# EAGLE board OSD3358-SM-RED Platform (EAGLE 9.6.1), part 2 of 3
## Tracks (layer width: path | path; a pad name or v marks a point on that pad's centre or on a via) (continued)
GND  (via drill 0.3, 0.3 pad 0.61, 0.5) (continued)
  Top 0.254: S1.4 S1.2 | S2.3 S2.1 | R37.2 v7.72,47.12 | R38.2 v7.72,49.02 | R35.2 v7.72,43.31 | R36.2 v7.72,45.21 | R26.2 v7.72,41.27 | X4.4 X4.8 | U14.4 17.53,7.42 17.37,7.26 v17.2,7.26 | U13.4 15.12,7.37 14.99,7.24 v14.61,7.24 | U11.4 18.79,15.38 18.92,15.24 R100.2 | C61.2 R100.2 | R100.2 v20.02,15.98 | C74.2 19.48,18.72 19.41,18.8 U12.4 | U12.4 | U12.4 18.79,18.29 18.67,18.16 v17.2,18.16 | C41.2 v21.79,16.64 | C40.2 v29.01,16.64 | C46.2 v25.43,22.12 | C2.1 70.32,10.93 v69.98,10.59 69.55,10.16 C1.1 | R59.1 R58.1 R56.1 R57.1 v81.56,46.43 | R65.1 R64.1 R63.1 R62.1 R61.1 R60.1 v86.54,45.54 | R66.1 R67.1 R68.1 v95.78,46.43 | R55.1 81.69,42.37 v81.25,42.37 | R54.1 R53.1 v83.19,45.06 | U10.61 U10.62 U10.63 87.05,41.17 v86.97,41.1 v91.59,41.1 91.55,41.14 U10.54 U10.53 | C14.2 C54.2 C59.2 96.11,28.78 v96.83,28.78 | R115.2 v26.04,35.56 | C57.2 C55.2 | C52.2 85.27,33.38 85.83,32.82 v85.93,32.72 | C62.2 v19.68,8.64 | v100.64,24.77 J4.8 | J4.10 v100.64,26.04 | J4.12 v100.64,27.3 | J4.16 v100.64,29.84 | J4.20 v100.64,32.38 | v100.64,22.23 J4.4 | C39.2 v93.12,27.03 93.12,27.48 93.03,27.57 Y3.2 | U7.N2 76.48,39.59 v76.48,38.43 | U7.G5 73.48,41.22 73.97,41.71 v74.37,41.71 | U7.J5 74.49,41.59 v74.37,41.71 | U7.E7 72.64,42.09 73.13,42.57 v73.13,42.98 73.56,42.98 73.99,43.41 U7.H10 | U7.K8 74.88,42.6 74.37,42.09 v74.37,41.71 | U7.A6 70.45,41.63 v69.47,41.63 | C91.2 85.83,24.61 v85.83,25.15 85.83,25.96 C89.2 | U22.9 U22.8 80.86,24.78 80.85,24.79 v79.88,24.79 79.4,24.79 C92.2 | v79.88,26.31 80.74,26.31 80.78,26.27 U22.5 | v82.78,26.57 82.73,26.52 82.45,26.52 82.2,26.27 U22.3
  Top 0.305: C93.2 v43.1,15.04 | v10.85,41.88 11.07,41.66 C3.2 | C51.2 v21.59,6.22 | U21.4 v38.48,10.54 | R39.1 v105.54,18.41 | C57.2 v96.83,30.86 | C21.2 95.38,17.65 v93.85,17.65 | C79.2 C88.2 v78.61,13.59
  Top 0.381: C22.2 v102.31,11.3 | C63.2 33.25,15.21 v33.86,15.21
  Top 0.762: D2.A 40.64,48.18 41.27,48.82 J5.1 | C11.- v35.56,36.35
  Bottom 0.152: R141.1 26.87,16.26 v26.49,15.88 | C13.1 v71.25,36.52 | X6.5 103.3,39.12 103.63,39.45 105.89,39.45 v106.05,39.29 | v103.66,40.59 103.45,40.59 103.18,40.32 X6.8 | X6.2 105.56,37.92 v106.07,38.43 | X6.16 100.5,38.52 v100.48,38.53 | v99.77,41 100,40.77 100,40.41 100.69,39.72 X6.13 | R18.1 54.86,27.91 55.09,27.69 v55.63,27.69 | 27.13,33.71 C77.2 C64.2 | C68.2 v24.92,27.05 | R1.2 43.54,35.03 v43.28,35.28 | C43.2 76.33,17.4 v76.58,17.14 | U2.4 10.42,47.02 v11.12,47.02 | U15.TH 25.04,18.69 v25.04,18.67 | v90.09,28.91 89.15,28.91 89.14,28.91 88.61,28.91 88.5,29.02 U25.1 | v55.63,26.42 55.3,26.75 R16.1
  Bottom 0.203: C75.2 v34.37,34.42 | C65.2 28.4,32.08 27.48,32.99 v27.1,32.99 | C78.2 v27.1,35.43 | C53.2 83.9,33.33 83.62,33.05 v83.62,32.82
  Bottom 0.254: v69.98,10.59 70.88,11.49 U6.1 72.38,11.49 72.67,11.79 R27.1 73.56,11.79 73.66,11.68 73.66,10.79 73.79,10.67 C6.1 | U6.4 74.05,9.99 74.22,10.16 C6.1 | C20.1 C18.1 73.28,48.11 73.43,48.26 v73.79,48.26 74.14,48.26 74.3,48.11 C19.1 | C35.2 C36.2 C37.2 C38.2 v80.85,31.55 | C34.2 C28.2 C27.2 | C27.2 C26.2 | C26.2 C25.2 | C32.2 C33.2 v86.97,41.1 C23.2 85.8,41.1 85.09,41.81 v85.09,42.6 | C31.2 C30.2 v91.59,41.1 92.35,41.1 C29.2 | C26.2 80.31,39.37 80.26,39.32 C24.2 79.86,39.29 v79.86,38.56 80.06,38.35 C27.2 | C77.2 C78.2 | C66.2 C67.2 25.98,32.74 26.24,32.99 v27.1,32.99 27.1,33.68 27.13,33.71 | C6.1 v74.98,10.67 | C17.1 75.41,41.71 v74.37,41.71 | C90.1 87.5,24.03 v88.06,24.59
  Bottom 0.305: R113.1 23.62,9.4 v24.13,9.91 | C16.1 v65.66,44.88 | X3.6 91.76,17.65 v93.85,17.65 | X3.GND 102.1,13.59 v101.22,13.59 | C101.2 C100.2 26.24,14.81 26.49,15.06 v26.49,15.88 | v24.89,10.67 24.89,9.65 24.64,9.4 C42.2 C99.2 | C50.2 26.67,9.45 26.21,9.91 v25.65,9.91 | 27.69,9.91 v27.18,9.91 | R112.1 27.69,9.91 | v27.18,11.43 27.74,10.87 C49.2 | R111.1 27.89,9.7 27.69,9.91
  Bottom 0.381: X1.GND v5.43,47.98 v5.44,47.98 | U15.1 28.66,20.02 28.83,20.19 28.83,20.83 v28.57,21.08 | v34.42,26.82 C76.2 C72.2 | v35.56,26.82 C70.2 C71.2
  other vias: 25.65,11.43 30.1,29.21 90.3,37.82 28.98,30.61 30.1,30.61 31.22,30.61 28.98,29.21 31.22,29.21 28.98,27.81 31.22,27.81 24.13,12.95 25.65,12.95 27.18,12.95 24.89,12.19 26.42,12.19 24.13,11.43 26.42,10.67 55.63,30.1 60.58,30.23 63.12,30.1 65.51,30.07 55.5,25.15 55.63,22.61 55.63,20.19 58.04,20.19 63.12,20.19 65.53,20.19 65.53,22.61 65.66,25.15 65.53,27.69 88.14,40.01 89.15,40.01 90.3,40.01 91.31,40.01 92.33,40.01 88.14,38.99 89.15,38.99 90.3,38.99 91.31,38.99 92.33,38.99 88.14,37.85 89.15,37.85 91.31,37.85 92.33,37.85 88.14,36.7 89.15,36.7 90.3,36.7 91.31,36.7 92.33,36.7 88.14,35.69 89.15,35.69 90.3,35.69 91.31,35.69 92.33,35.69 30.1,27.81 25.04,19.43 25.81,19.43 25.81,18.67 33.86,15.98 86.79,32.69 99.19,36.83 99.24,40.36 85.17,37.82 80.85,29.77 60.58,20.19 48.16,41 48.16,38.89 49.23,37.8 43.56,37.97 19.05,47.5 19.05,48.39 19.05,46.61 24,48.39 24,47.5 24,46.61 59.74,42.52 59.74,41.76 56.77,20.19 59.31,20.19 61.85,20.19 64.26,20.19 65.53,23.88 61.85,30.1 64.39,30.1
  pour Route2: -3.81,58.42 111.76,58.42 111.76,-3.81 -3.81,-3.81
  pour Top (rank 6): 55.5,20.07 59.31,20.07 59.31,19.43 61.85,19.43 61.85,20.07 65.66,20.07 65.66,23.88 66.29,23.88 66.29,26.42 65.66,26.42 65.66,30.23 61.85,30.23 61.85,30.86 59.31,30.86 59.31,30.23 55.5,30.23 55.5,26.42 54.86,26.42 54.86,23.88 56.13,23.88 56.13,29.59 65.02,29.59 65.02,20.7 56.13,20.7 56.13,23.24 55.5,23.24
  pour Top (rank 6): 55.5,23.24 55.5,23.88 56.13,23.88 56.13,23.24
  pour Top: 19.94,45.09 17.78,47.24 15.88,47.24 15.37,46.74 13.59,46.74 13.21,47.12 13.21,48.39 17.91,48.39 18.41,48.9 24.13,48.9 24.77,48.26 24.77,45.72 24.13,45.09
  pour Top (no thermals): 85.6,34.16 87.25,34.16 87.63,33.78 87.63,32.72 87.05,32.13 85.47,32.13 85.22,32.38 85.22,33.66
  pour Top (no thermals): 85.72,38.3 86.39,38.3 86.39,37.41 84.84,37.41 84.84,38.3
  pour Top (no thermals): 86.87,42.57 88.24,42.57 88.24,40.64 87,40.64 86.87,40.64 86.56,40.94 86.56,41.48 86.87,41.78
  pour Top (no thermals): 91.72,42.57 92.28,42.57 92.28,40.64 91.29,40.64 91.29,42.57
  pour Bottom (no thermals): 81.38,29.31 80.62,29.31 80.62,30.18 81.41,30.18 81.41,31.22 80.62,31.22 80.62,31.8 82.04,31.8 82.04,29.87 81.94,29.87
  pour Bottom (no thermals): 30.35,16.76 34.16,16.76 34.16,13.59 31.11,13.59 31.11,14.61 30.35,14.61
  pour Top (no thermals): 96.85,40.31 98.78,40.31 99.14,40.67 99.62,40.67 99.62,40.11 98.6,40.11 98.42,39.93 96.85,39.93
  pour Top (no thermals): 96.88,37.24 99.69,37.19 99.69,36.53 99.14,36.53 98.91,36.83 96.88,36.83
  pour Top (no thermals): 89,28.5 89,29.51 90.4,29.51 90.4,28.24 89.76,28.24 89.76,29.21 89.76,29.24 89.26,29.24 89.26,28.5
  pour Top (rank 2, no thermals): 50.14,39.62 48.46,39.62 48.46,38.56 49.53,38.56 49.53,37.64 50.29,37.64 50.29,36.73 49.07,36.73 49.07,38.1 48.16,38.1 47.7,38.71 47.7,41.76 48.46,41.76 48.46,40.23 50.14,40.23
  pour Top (rank 2, no thermals): 43.18,38.73 44.83,38.73 44.83,37.21 43.18,37.21
  pour Bottom: 18.54,48.64 24.38,48.64 24.38,45.09 18.54,45.09
  pour Top (no thermals): 57.91,42.82 61.72,42.82 61.72,41.45 57.91,41.45
GPIO0_7  (via drill 0.3)
  Top 0.152: v79.27,15.04 79.07,15.24 R9.2 77.98,15.24 77.85,15.37 77.85,16.64 v77.34,17.14
  Bottom 0.152: v79.27,15.04 79.88,14.43 80.97,14.43 84.58,10.82 84.58,9.75 85.5,8.84 85.5,6.86 86.56,5.79 90.73,5.79 J6.42 | R2.2 76.66,18.49 77.34,17.8 v77.34,17.14
GPIO0_7SRC  (via drill 0.3)
  Top 0.152: U1.C5 64.59,18.16 64.39,17.96 v64.39,17.3
  Bottom 0.152: v64.39,17.3 64.39,17.02 64.62,16.79 65.15,16.79 65.89,17.53 71.07,17.53 72.03,18.49 R2.1
GPIO0_26  (via drill 0.3)
  Top 0.152: U1.R5 65.02,33.96 65.51,34.44 65.51,35.36 64.77,36.09 64.77,45.97 62.69,48.06 62.69,50.8 62.48,51 v62.48,51.44
  Bottom 0.152: J5.14 56.52,51.94 56.87,51.59 61.9,51.59 62.05,51.44 v62.48,51.44
GPIO0_27
  Top 0.152: U1.T5 65.02,35.41 64.47,35.97 64.47,45.85 61.59,48.72 J5.17
GPIO1_12
  Top 0.152: U1.P6 63.75,32.64 62.97,33.43 62.97,35.31 62.94,35.33 62.94,45.21 61.52,46.63 60.07,46.63 58.24,48.46 54.13,48.46 52.91,49.68 52.91,51.64 J5.12
GPIO1_13
  Top 0.152: U1.R6 63.27,33.88 63.27,35.43 63.25,35.46 63.25,45.34 61.65,46.94 60.2,46.94 58.37,48.77 55.37,48.77 J5.11
GPIO1_14
  Top 0.152: U1.T6 63.75,35.38 63.55,35.59 63.55,45.47 61.77,47.24 60.33,47.24 57.96,49.61 57.96,51.61 J5.16
GPIO1_15
  Top 0.152: U1.P7 62.97,31.65 63.96,31.65 64.24,31.93 64.24,35.33 63.86,35.71 63.86,45.59 61.9,47.55 60.45,47.55 59.05,48.95 J5.15
GPIO1_16
  Bottom 0.152: R14.2 R23.2 56.03,32.26 55.78,32 55.02,32 53.24,30.23 52.88,30.23 52.4,29.74 52.4,24.28 50.37,22.25 50.37,15.34 52.83,12.88 52.83,7.11 53.7,6.25 58.83,6.25 60.2,4.88 60.2,3.05 J6.15
GPIO1_17  (via drill 0.3)
  Top 0.152: U1.R12 56.13,32.82 56.62,32.33 56.62,31.93 56.16,31.47 v55.75,31.47
  Bottom 0.152: v55.75,31.47 54.91,31.47 53.37,29.92 53.01,29.92 52.7,29.62 52.7,24.16 50.67,22.12 50.67,15.47 53.14,13.01 53.14,7.24 53.82,6.55 58.95,6.55 60.5,5 60.5,3.5 60.96,3.05 62.2,3.05 62.87,2.39 62.87,1.27 63.3,0.84 68.15,0.84 J6.23
GPIO1_28  (via drill 0.3)
  Top 0.152: U1.N14 53.59,31.45 53.44,31.6 v52.98,31.6
  Bottom 0.152: v52.98,31.6 52.96,31.6 51.49,30.12 51.49,24.66 49.45,22.63 49.45,14.96 51.92,12.5 51.92,6.5 J6.12
GPIO1_29  (via drill 0.3)
  Top 0.152: U1.P3 68.15,32.13 68.63,32.61 70.43,32.61 73.28,35.46 v73.28,35.97
  Bottom 0.152: v73.28,35.97 73.28,38.84 69.98,42.14 69.98,44.55 69.32,45.21 69.32,45.87 69.47,46.02 69.47,47.99 70.64,49.16 70.64,52.48 70.87,52.7 J5.26
GPIO2_1  (via drill 0.3)
  Top 0.152: U1.T7 62.48,35.36 62.64,35.51 62.64,44.96 61.27,46.33 59.89,46.33 58.67,47.55 v58.06,47.55
  Bottom 0.152: v58.06,47.55 62.15,47.55 63.07,48.46 63.07,52.22 62.59,52.7 J5.18
GPIO3_18  (via drill 0.3)
  Top 0.152: U1.A3 67.67,15.62 68.68,14.61 69.57,14.61 70.21,13.97 v70.21,13.64 | R9.1 77.29,14.71 77.03,14.44 73.6,14.44 73.38,14.22 v73.18,14.22
  Bottom 0.152: v70.21,13.64 70.41,13.44 72.36,13.44 73.15,14.22 v73.18,14.22
GPIO3_19
  Top 0.152: U1.B3 67.56,16.33 68.05,15.85 68.05,15.72 68.83,14.94 69.67,14.94 71.12,13.49 71.12,9.09 70.56,8.53 70.56,6.55 71.32,5.79 72.54,5.79 73.15,5.18 73.15,3.05 J6.27
GPIO3_20
  Top 0.152: R7.1 69.47,13.99 69.16,14.3 68.56,14.3 67.77,15.09 67.41,15.09 67.08,15.42 67.08,17.17 67.56,17.65 U1.C3
GPIO3_21
  Top 0.152: R114.2 72.39,15.44 72.14,15.7 72.14,16.54 71.3,17.37 68.43,17.37 68.05,17.75 68.05,18.52 67.82,18.75 67.26,18.75 66.67,18.16 U1.C4 65.89,18.16 65.66,17.93 65.66,15.47 66.62,14.5 66.62,11.15 66.42,10.95 66.42,9.53 66.95,8.99 69.37,8.99 70.26,8.1 70.26,6.4 71.17,5.49 72.39,5.49 72.85,5.03 72.85,3 J6.25
HDMI_CEC  (via drill 0.3)
  Top 0.152: U10.30 93.05,33.17 93.8,32.41 94.61,32.41 v95.35,31.67 94.59,31.67 93.65,30.73 93.65,25.25 93.07,24.67 D11.C
  Bottom 0.152: X6.12 100.73,40.12 100.31,40.54 100.31,41.78 99.9,42.19 98.15,42.19 97.79,41.83 97.79,32.56 97.43,32.21 95.89,32.21 v95.35,31.67
HDMI_CEC_D
  Top 0.152: R140.2 94.08,23.39 93.11,22.42 D11.A
HDMI_CLK_INH  (via drill 0.3)
  Top 0.152: v88.9,19.43 88.9,20.07 88.29,20.68 88.29,23.04 88.95,23.7 89.94,23.7 90.7,24.46 90.7,26.82 90.91,27.03 R110.1 91.26,28.19 Y3.1 | v88.54,12.5 88.54,11.89 87.94,11.28 86.59,11.28 85.95,10.64 85.95,8.23 85.34,7.62 J7.1
  Bottom 0.152: v88.9,19.43 88.88,19.41 88.88,12.83 v88.54,12.5
HDMI_DSCL  (via drill 0.3)
  Top 0.152: U10.33 94.65,33.77 95.15,33.27 96.39,33.27 96.57,33.1 v96.95,33.1 | v99.34,42.72 98.63,43.43 98.63,44.6 v98.83,44.81
  Bottom 0.152: v96.95,33.1 97.13,33.27 97.13,33.68 97.48,34.04 97.48,42.6 98.15,43.26 99.62,43.26 100.13,42.75 | X6.11 100.76,40.52 100.61,40.66 100.61,42.27 100.38,42.49 | 100.38,42.49 100.13,42.75 | 100.38,42.49 100.13,42.49 | 100.13,42.49 99.57,42.49 v99.34,42.72 | R147.1 97.46,45.49 97.74,45.21 98.65,45.21 98.83,45.03 v98.83,44.81 | 100.13,42.75 100.13,42.49
HDMI_DSDA  (via drill 0.3)
  Top 0.152: U10.32 94.47,33.47 95.2,32.74 v96.09,32.74
  Bottom 0.152: v96.09,32.74 96.32,32.74 96.39,32.82 96.39,33.38 97.18,34.16 97.18,42.72 98.02,43.56 99.47,43.56 | X6.9 102.11,40.72 102.06,40.77 102.06,41.12 101.85,41.33 101.85,41.88 101.68,42.06 101.24,42.06 99.75,43.56 99.64,43.56 | 99.64,43.56 99.47,43.56 | R148.1 98.42,46.1 99.69,44.83 99.69,43.79 | 99.69,43.79 99.69,43.61 99.64,43.56 | 99.47,43.56 99.69,43.79
HDMI_HPD  (via drill 0.3)
  Top 0.152: U10.31 93.55,33.12 93.95,32.72 94.79,32.72 95.07,32.44 95.45,32.44 v96.22,31.67
  Bottom 0.152: X6.19 100.51,37.32 100.25,37.06 99.97,37.06 99.75,36.83 99.75,36.47 99.57,36.3 98.42,36.3 98.2,36.07 98.2,32.44 97.43,31.67 v96.22,31.67
HDMI_INT  (via drill 0.3, 0.3 pad 0.61)
  Top 0.152: U10.50 93.55,42.59 94.08,43.13 96.09,43.13 96.5,43.54 R130.1 96.5,46.89 96.39,46.99 95.91,46.99 95.78,47.12 95.78,48.59 96.09,48.9 97.54,48.9 98.22,49.58 98.22,51.08 v97.99,51.31 | U1.T15 52.02,34.67 v51.69,35 | v75.54,35.97 76.05,35.97 76.53,36.45 77.19,36.45 79.02,38.28 79.02,41.53 78,42.55 78,51.31 v77.78,51.54
  Bottom 0.152: v77.78,51.54 97.77,51.54 v97.99,51.31 | v75.54,35.97 75.54,34.09 75.87,33.76 71.14,29.03 69.27,29.03 68.89,28.65 67.69,28.65 65.23,31.11 65.23,32.03 62.33,34.92 58.85,34.92 58.42,35.36 58.42,36.52 56.59,38.35 51.71,38.35 51.51,38.15 51.51,35.18 v51.69,35
HDMI_SWING
  Top 0.152: U10.34 95.53,34.57 95.71,34.39 95.71,34.19 95.91,33.98 R136.2
HDMI_TX0+  (via drill 0.3)
  Top 0.152: U10.40 95.07,37.57 95.15,37.49 95.73,37.49 95.89,37.64 95.89,38.56 96.01,38.68 96.27,38.68 96.39,38.56 96.39,38.02 96.52,37.9 96.65,37.9 96.75,38 97.14,38 D9.5 97.84,38.01 D9.6 98.31,38.01 98.42,37.9 98.83,37.9 v99.14,38.2
  Bottom 0.152: X6.15 100.89,38.92 100.74,39.06 100.23,39.06 99.59,38.43 99.36,38.43 v99.14,38.2
HDMI_TX0-  (via drill 0.3)
  Top 0.152: U10.39 95.03,37.07 95.15,37.19 95.86,37.19 96.27,37.59 96.65,37.59 96.73,37.51 D9.4 97.84,37.51 D9.7 98.31,37.51 98.4,37.59 99.39,37.59 99.67,37.87 99.67,38.43 v99.14,38.96
  Bottom 0.152: v99.14,38.96 99.36,38.73 99.47,38.73 100.1,39.37 100.86,39.37 100.92,39.32 X6.14
HDMI_TX1+  (via drill 0.3)
  Top 0.152: U10.43 95.17,39.07 95.28,38.96 95.4,38.96 95.96,39.52 96.65,39.52 96.76,39.63 D8.2 97.84,39.63 D8.9 98.31,39.63 98.4,39.55 98.5,39.55 98.75,39.8 103.94,39.8 104.62,39.12 v104.62,38.89
  Bottom 0.152: X6.3 103.19,38.32 103.25,38.38 104.11,38.38 v104.62,38.89
HDMI_TX1-  (via drill 0.3)
  Top 0.152: U10.42 95.14,38.57 95.22,38.66 95.53,38.66 96.09,39.22 96.67,39.22 96.76,39.13 D8.1 97.84,39.13 D8.10 98.31,39.13 98.4,39.22 98.63,39.22 98.91,39.5 100.97,39.5 101.09,39.37 101.09,38.61 101.22,38.48 101.6,38.48 101.73,38.61 101.73,39.37 101.85,39.5 103.66,39.5 103.86,39.29 v103.86,38.91
  Bottom 0.152: X6.4 103.17,38.72 103.2,38.68 103.63,38.68 v103.86,38.91
HDMI_TX2+  (via drill 0.3)
  Top 0.152: U10.45 95.21,40.07 95.3,39.98 95.56,39.98 95.71,40.13 95.71,40.62 96.11,41.02 96.65,41.02 96.76,41.13 D8.5 D8.6 98.29,41.13 98.4,41.02 98.65,41.02 98.81,41.17 98.81,41.43 v98.58,41.66
  Bottom 0.152: v98.58,41.66 98.22,41.3 98.22,37.72 98.58,37.36 100.13,37.36 100.46,37.69 100.81,37.69 100.83,37.72 X6.18
HDMI_TX2-  (via drill 0.3)
  Top 0.152: U10.44 95.17,39.57 95.28,39.67 95.68,39.67 96.01,40.01 96.01,40.49 96.24,40.72 96.65,40.72 96.73,40.63 D8.4 D8.7 97.99,40.63 98.29,40.63 98.37,40.72 98.81,40.72 99.11,41.02 99.11,41.4 v99.34,41.63
  Bottom 0.152: X6.17 100.83,38.12 100.71,38 100.33,38 100,37.67 98.7,37.67 98.53,37.85 98.53,40.82 v99.34,41.63
HDMI_TXC+  (via drill 0.3)
  Top 0.152: U10.38 95.05,36.57 95.12,36.5 96.14,36.5 96.24,36.4 96.65,36.4 96.76,36.51 D9.2 D9.9 | v104.57,39.98 105.16,39.4 105.16,38.43 105,38.28 103.89,38.28 103.4,37.8 103.4,36.73 102.97,36.3 100.74,36.3 100.58,36.45 100.58,37.21 100.46,37.34 100.08,37.34 99.95,37.21 99.95,36.45 99.8,36.3 98.93,36.3 98.83,36.4 98.45,36.4 98.35,36.5 D9.9 | D9.9
  Bottom 0.152: X6.6 103.25,39.52 103.48,39.75 104.01,39.75 104.24,39.98 v104.57,39.98
HDMI_TXC-  (via drill 0.3)
  Top 0.152: U10.37 95,36.07 95.12,36.2 95.96,36.2 96.06,36.09 96.65,36.09 96.75,35.99 97.14,35.99 D9.1 D9.10 98.31,36.01 98.4,36.09 98.7,36.09 98.81,35.99 103.2,35.99 103.71,36.5 103.71,37.64 104.04,37.97 105.21,37.97 105.46,38.23 105.46,39.85 v105.33,39.98
  Bottom 0.152: X6.7 103.21,39.92 103.35,40.06 103.89,40.06 104.34,40.51 104.8,40.51 v105.33,39.98 | X6.7
HDMICLK_DISN  (via drill 0.3)
  Top 0.152: Y5.1 75.11,14.76 72.85,14.76 72.64,14.55 72.64,10.46 73.51,9.6 77.52,9.6 78.11,9.02 78.11,3.73 78.79,3.05 79.86,3.05 80.47,2.44 80.47,1.29 80.01,0.84 45.57,0.84 45.06,1.35 v45.06,2.41 | U1.T16 48.84,34.67 48.23,35.28 v44.04,35.28
  Bottom 0.152: v45.06,2.41 45.06,4.75 42.75,7.06 42.75,8.66 43.64,9.55 43.64,18.24 45.97,20.57 45.97,28.55 44.2,30.33 44.2,34.14 44.04,34.29 v44.04,35.28
I2C0_SCL  (via drill 0.3, 0.3 pad 0.61)
  Top 0.152: U1.D10 U1.C10 59.46,18.95 66.52,18.95 66.78,19.2 66.78,19.91 67.08,20.22 74.27,20.22 74.6,19.89 v74.95,19.89 76.4,19.89 78.33,21.82 81.97,21.82 82.7,22.55 82.7,23.77 v82.5,23.98 83.31,24.79 83.31,25.78 83.06,26.04 82.43,26.04 82.17,25.78 U22.2 | U17.D4 90.74,15.33 90.07,16 87.05,16 84.3,18.75 83.06,18.75 v82.75,18.44 82.75,17.68 82.83,17.6 R12.1 82.83,16.89 82.42,16.48 82.42,16.26 82.48,16.2 U16.29 | v95.45,44.83 95.22,44.6 93.6,44.6 92.66,43.66 92.66,42.57 92.55,42.46 U10.52 | v91.75,32.16 91.75,31.7 90.53,30.48 v90.53,30.02 | J15.1 80.64,8.56 80.77,8.69 84.28,8.69 85.19,9.6 v85.19,10.06
  Bottom 0.152: v95.45,44.83 95.68,44.6 95.99,44.6 96.24,44.35 96.24,34.52 94.34,32.61 92.2,32.61 v91.75,32.16 | v74.95,19.89 76.33,19.89 76.73,20.3 79.05,20.3 80.29,19.05 81.69,19.05 82.3,18.44 v82.75,18.44 83.06,18.75 83.82,18.75 84.12,18.44 84.12,13.26 85.8,11.58 85.8,10.67 v85.19,10.06 | U25.6 90.04,29.94 90.12,30.02 v90.53,30.02 90.53,30.94 90.22,31.24 86.92,31.24 85.78,30.1 85.78,29.29 85.7,29.21 85.52,29.21 85.32,29.41 85.09,29.41 84.89,29.21 84.89,29.01 85.09,28.8 85.09,28.3 84.51,27.71 84.51,27.15 84.4,27.05 84.15,27.05 84.02,26.92 84.02,26.54 84.12,26.44 84.4,26.44 84.51,26.34 84.51,24.84 84.18,24.51 82.91,24.51 82.5,24.11 v82.5,23.98
I2C0_SCL_1P8V  (via drill 0.3)
  Top 0.152: U23.23 87.92,29.1 87.68,29.34 87.1,29.34 v86.94,29.18
  Bottom 0.152: U25.3 88.04,29.94 88.04,29.95 87.25,29.95 86.94,29.64 v86.94,29.18 86.94,28.63 86.56,28.25 86.56,27.36 R163.1
I2C0_SDA  (via drill 0.3, 0.3 pad 0.61)
  Top 0.152: U1.D11 U1.C11 57.94,18.16 58.42,17.68 59.21,17.68 59.41,17.88 59.41,18.44 59.61,18.64 66.65,18.64 67.08,19.07 67.08,19.71 67.28,19.91 74.12,19.91 74.32,19.71 v74.32,19.43 74.4,19.36 75.21,19.36 75.44,19.58 76.56,19.58 78.49,21.51 82.14,21.51 83.01,22.38 83.01,23.75 83.24,23.98 v83.26,23.98 83.59,24.31 83.59,26.77 83.19,27.18 81.79,27.18 81.41,26.8 U22.4 | U17.C4 90.68,14.93 89.92,15.7 86.92,15.7 84.48,18.14 v83.52,18.14 | U10.51 93.05,42.49 92.96,42.57 92.96,43.54 93.73,44.3 95.22,44.3 v95.45,44.07 | U16.30 82.08,16.19 82.12,16.23 82.12,16.46 81.71,16.87 R13.1 81.71,17.5 81.84,17.63 v81.84,18.14 | v89.92,30.63 91.08,31.8 v91.08,32.61 | J15.2 80.64,9.12 80.77,8.99 84.12,8.99 84.58,9.45 84.58,10.21 v85.19,10.82
  Bottom 0.152: v95.45,44.07 95.94,43.59 95.94,34.65 94.21,32.92 91.39,32.92 v91.08,32.61 | v74.32,19.43 74.4,19.36 75.21,19.36 75.44,19.58 76.45,19.58 76.86,19.99 78.92,19.99 80.16,18.75 81.23,18.75 v81.84,18.14 82.14,17.83 83.21,17.83 v83.52,18.14 83.82,17.83 83.82,13.11 85.19,11.73 v85.19,10.82 | U25.5 89.36,30.3 89.74,30.3 89.92,30.48 v89.92,30.63 89.61,30.94 87.05,30.94 86.08,29.97 86.08,28.85 84.81,27.58 84.81,24.41 84.48,24.08 83.36,24.08 v83.26,23.98
I2C0_SDA_1P8V  (via drill 0.3)
  Top 0.152: U23.24 87.48,28.8 87.33,28.65 86.39,28.65 85.95,28.22 v85.95,27.94
  Bottom 0.152: R164.1 85.32,27.56 85.5,27.74 85.83,27.74 85.95,27.86 v85.95,27.94 85.95,28.22 86.39,28.65 86.39,29.79 86.89,30.29 U25.4
I2C1_SCL
  Top 0.152: U18.B2 38.08,15.47 38.08,16.31 37.72,16.66 36.42,16.66 R154.2 36.3,16.54 35.87,16.54 35.23,15.9 35.23,7.62 36.14,6.71 38.3,6.71 39.73,5.28 39.73,3.53 40.21,3.05 60.45,3.05 J6.17
I2C1_SCL_COMB  (via drill 0.3 pad 0.61)
  Top 0.152: U18.A1 37.05,15.44 R154.1 36.3,15.47 36.27,15.44 35.97,15.44 35.79,15.27 v35.79,14.61 | v38.71,15.65 38.71,15.95 38.99,16.23 47.7,16.23 49.45,14.48 52.45,14.48 U1.A14
  Bottom 0.152: v38.71,15.65 38.2,15.14 36.32,15.14 v35.79,14.61
I2C1_SDA
  Top 0.152: U20.B2 46.74,9.27 46.74,8.51 47.02,8.23 48.54,8.23 R159.2 53.7,8.33 54.25,7.77 54.25,6.25 55.02,5.49 60.55,5.49 J6.18
I2C1_SDA_COMB
  Top 0.152: U20.A1 47.91,9.45 R159.1 54.59,9.45 55.35,10.21 55.35,17.12 55.04,17.42 54.13,17.42 U1.B14
I2C2_SCL  (via drill 0.3)
  Top 0.152: U1.A10 58.67,14.81 57.76,13.89 v57.76,11.58
  Bottom 0.152: J6.19 62.99,3.05 62.99,5.16 62.03,6.12 62.03,6.55 57.99,10.59 57.99,11.35 v57.76,11.58
I2C2_SDA  (via drill 0.3)
  Top 0.152: U1.B10 58.7,16.89 59.16,16.43 59.16,14.86 58.29,13.99 v58.29,12.19
  Bottom 0.152: J6.20 62.33,6.25 62.33,6.71 58.29,10.74 v58.29,12.19
IMU_INT  (via drill 0.3)
  Top 0.152: U1.E15 51.99,21.03 v51.74,21.03 | v86.64,23.7 88.49,23.7 89.18,24.38 89.18,25.17 89.52,25.51 U23.12
  Bottom 0.152: v51.74,21.03 52.43,21.03 52.73,20.73 65.84,20.73 66.24,20.32 67.31,20.32 67.67,20.68 67.67,23.5 70.46,26.29 76.73,26.29 76.94,26.09 76.94,24.77 77.75,23.95 80.57,23.95 81.81,22.71 85.75,22.71 86.11,23.06 86.11,23.34 86.46,23.7 v86.64,23.7
JTAG_EMU0  (via drill 0.3, 0.3 pad 0.61)
  Top 0.152: U1.E2 69.32,21.18 70.66,21.18 73.97,24.49 v75.01,24.49 | J4.13 102.23,28.57 101.6,27.94 97.28,27.94 97.08,27.74 97.08,25.63 96.44,24.99 96.19,24.99 96.06,24.87 R40.1 95.66,24.46 95.5,24.31 95.5,24.05 95.38,23.93 93.9,23.93 93.4,23.42 90.53,23.42 89.97,22.86 v89.38,22.86
  Bottom 0.152: v75.01,24.49 76.78,24.49 77.62,23.65 80.44,23.65 81.69,22.4 88.14,22.4 88.59,22.86 v89.38,22.86
JTAG_EMU1  (via drill 0.3)
  Top 0.152: U1.E3 67.97,21.11 v68.2,21.11 | J4.14 97.38,28.57 96.77,27.96 96.77,25.78 96.52,25.53 R41.1 95.63,25.53 95.5,25.4 95.5,25.12 95.38,24.99 93.88,24.99 93.65,24.77 93.65,24.36 93.02,23.72 90.4,23.72 90.07,23.39 89.1,23.39 88.82,23.11 v88.82,22.33
  Bottom 0.152: v68.2,21.11 71.2,21.11 73.71,23.62 77.22,23.62 77.5,23.34 80.31,23.34 81.56,22.1 88.59,22.1 v88.82,22.33
JTAG_TCK
  Top 0.152: J4.11 J4.9 101.98,26.04 101.35,25.4 97.28,25.4 96.72,24.84 96.72,23.16 95.22,21.67 93.12,21.67 89.79,18.34 88.09,18.34 86.13,20.3 81.41,20.3 80.01,18.9 71.17,18.9 70.64,19.43 U1.D1
JTAG_TDI
  Top 0.152: U1.C1 70.28,17.98 80.39,17.98 81.79,19.38 85.75,19.38 87.71,17.42 90.17,17.42 93.5,20.75 95.61,20.75 96.44,21.59 101.22,21.59 102.62,20.19 105.66,20.19 105.87,20.4 105.87,22.02 105.66,22.23 J4.3
JTAG_TDO
  Top 0.152: U1.C2 69.32,18.64 70.54,18.64 70.89,18.29 80.26,18.29 81.66,19.68 85.88,19.68 87.83,17.73 90.04,17.73 93.37,21.06 95.48,21.06 97.28,22.86 100.38,22.86 102.29,24.77 J4.7
JTAG_TMS
  Top 0.152: U1.D2 69.32,18.95 70.66,18.95 71.02,18.59 80.14,18.59 81.53,19.99 86,19.99 87.96,18.03 89.92,18.03 93.24,21.36 95.35,21.36 97.03,23.04 97.03,23.85 97.31,24.13 101.09,24.13 102.36,25.4 105.64,25.4 105.87,25.17 105.87,23.09 105.64,22.86 102.49,22.86 102.23,22.61 102.23,21.21 102.49,20.95 J4.1
JTAG_TRSTN
  Top 0.152: U1.D3 68.35,18.64 68.35,17.88 68.56,17.68 80.52,17.68 81.92,19.07 85.62,19.07 87.58,17.12 90.3,17.12 93.62,20.45 95.73,20.45 96.24,20.95 J4.2 101.37,20.95 103.45,18.87 R39.2
LCD_DATA0  (via drill 0.3)
  Top 0.152: R68.2 v95.07,48.36 96.88,50.16 J5.45 | U1.G3 68.07,23.24 68.86,22.45 70.61,22.45 82.42,34.27 v84.3,34.27 84.56,34.52 85.52,34.52 85.57,34.57 U10.15
  Bottom 0.152: v95.07,48.36 R85.1 96.01,47.42 96.88,46.56 96.88,34.29 94.59,32 93.02,32 92.25,31.24 91.16,31.24 90.55,31.85 85.5,31.85 84.91,32.44 84.91,33.66 v84.3,34.27 82.3,32.26 C38.1
LCD_DATA1  (via drill 0.3)
  Top 0.152: R67.2 v94,48.36 94.61,48.97 95.02,48.97 95.68,49.63 95.68,51.23 J5.46 | U1.G2 69.32,23.24 69.8,22.76 70.48,22.76 82.75,35.03 v84.3,35.03 84.89,35.61 85.52,35.61 85.56,35.57 U10.13
  Bottom 0.152: v94,48.36 R84.1 94,47.04 94.18,46.86 95.43,46.86 95.53,46.97 96.04,46.97 96.55,46.46 96.55,34.39 94.46,32.31 92.89,32.31 92.13,31.55 91.29,31.55 90.68,32.16 85.62,32.16 85.22,32.56 85.22,34.29 84.48,35.03 v84.3,35.03 82.55,33.27 C37.1
LCD_DATA2  (via drill 0.3)
  Top 0.152: U1.G1 70.54,23.24 83.08,35.79 v84.28,35.79 84.56,36.07 U10.12 | R66.2 v92.94,48.36 92.94,48.49 J5.43 | R69.1 98.44,48.22 v98.27,48.39
  Bottom 0.152: v92.94,48.36 R83.1 92.94,46.99 93.07,46.86 93.34,46.86 93.47,46.74 93.47,45.34 94.74,44.07 94.74,34.54 93.45,33.25 87.07,33.25 85.72,34.59 85.72,35.41 85.06,36.07 84.56,36.07 v84.28,35.79 82.78,34.29 C36.1 | J5.43 95.68,49.1 97.56,49.1 v98.27,48.39
LCD_DATA3  (via drill 0.3)
  Top 0.152: U10.11 84.3,36.57 v84.28,36.55 83.41,36.55 70.59,23.72 68.35,23.72 U1.H3 | J5.44 93.14,51.23 93.14,49.63 v91.87,48.36 R65.2 91.87,47.07 91.97,46.97 92.28,46.97 92.41,46.84 92.41,45.77 v92.63,45.54
  Bottom 0.152: v91.87,48.36 R82.1 | v92.63,45.54 92.84,45.54 94.44,43.94 94.44,34.67 93.32,33.55 87.2,33.55 86.03,34.72 86.03,35.87 85.32,36.58 84.3,36.58 v84.28,36.55 83.03,35.31 C35.1
LCD_DATA4  (via drill 0.3)
  Top 0.152: R64.2 v90.81,48.36 90.81,48.9 J5.41 | U10.10 84.52,37.07 v84.28,37.31 83.74,37.31 70.46,24.03 69.32,24.03 U1.H2
  Bottom 0.152: v90.81,48.36 R81.1 90.81,46.97 90.91,46.86 91.24,46.86 91.34,46.76 91.34,45.31 91.64,45.01 92.94,45.01 94.13,43.81 94.13,34.8 93.19,33.86 87.33,33.86 86.33,34.85 86.33,36.32 85.57,37.08 84.51,37.08 v84.28,37.31 83.29,36.32 C34.1
LCD_DATA5  (via drill 0.3)
  Top 0.152: U1.H1 70.51,24.51 84.07,38.08 v84.25,38.08 84.75,38.57 U10.7 | R63.2 v89.74,48.36 90.6,49.23 90.6,51.23 J5.42
  Bottom 0.152: v89.74,48.36 R80.1 89.74,46.99 89.86,46.86 90.12,46.86 90.27,46.71 90.27,45.24 90.81,44.7 92.81,44.7 93.83,43.69 93.83,34.92 93.07,34.16 87.45,34.16 86.64,34.98 86.64,37.82 85.88,38.58 84.76,38.58 v84.25,38.08 83.52,37.34 C28.1
LCD_DATA6  (via drill 0.3)
  Top 0.152: R62.2 v88.67,48.36 88.67,49.3 J5.39 | U1.J3 68.35,24.99 70.56,24.99 83.08,37.52 83.08,38.33 83.62,38.86 v84.28,38.86 84.43,39.01 85.37,39.01 85.43,39.07 U10.6
  Bottom 0.152: v88.67,48.36 R79.1 88.67,46.99 88.8,46.86 89.08,46.86 89.2,46.74 89.2,45.29 90.09,44.4 92.69,44.4 93.52,43.56 93.52,35.05 92.94,34.47 87.58,34.47 86.94,35.1 86.94,38.35 86.26,39.04 84.45,39.04 v84.28,38.86 83.77,38.35 C27.1
LCD_DATA7  (via drill 0.3)
  Top 0.152: R61.2 v87.61,48.36 88.06,48.82 88.06,51.23 J5.40 | U10.3 84.8,40.57 v84.25,41.12 82.78,39.65 82.78,37.64 70.43,25.3 69.32,25.3 U1.J2
  Bottom 0.152: v87.61,48.36 R78.1 87.61,46.97 87.71,46.86 88.01,46.86 88.14,46.74 88.14,45.31 89.36,44.09 92.56,44.09 93.22,43.43 93.22,35.18 92.81,34.77 87.71,34.77 87.25,35.23 87.25,39.29 86.28,40.26 85.11,40.26 v84.25,41.12 82.5,39.37 C26.1
LCD_DATA8  (via drill 0.3)
  Top 0.152: U1.J1 70.48,25.78 82.47,37.77 82.47,40.13 v84.25,41.91 85.09,41.07 U10.2 | R60.2 v86.54,48.36 87,48.82 J5.37
  Bottom 0.152: v86.54,48.36 R77.1 86.54,46.97 86.64,46.86 86.94,46.86 87.07,46.74 87.07,45.24 87.38,44.93 87.55,44.93 88.7,43.79 92.43,43.79 92.91,43.31 92.91,35.31 92.69,35.08 87.83,35.08 87.55,35.36 87.55,39.42 86.41,40.56 85.6,40.56 v84.25,41.91 82.73,40.39 C25.1
LCD_DATA9  (via drill 0.3)
  Top 0.152: R59.2 v85.47,48.36 85.47,49 85.93,49.45 85.93,51.64 J5.38 | U10.1 85.35,41.57 v84.25,42.67 82.17,40.59 82.17,37.9 70.54,26.26 68.35,26.26 U1.K3
  Bottom 0.152: R76.1 v85.47,48.36 85.7,48.59 85.7,50.62 85.09,51.23 81.18,51.23 80.62,50.67 80.62,49.55 80.16,49.1 79.3,49.1 77.47,47.27 77.47,43.94 79.98,41.43 | v84.25,42.67 82.5,40.92 80.49,40.92 80.14,41.27 | 80.14,41.27 79.98,41.43 | C24.1 79.83,41.27 | 79.83,41.27 79.98,41.43 | 79.83,41.27 80.14,41.27
LCD_DATA10  (via drill 0.3)
  Top 0.152: R58.2 v84.4,48.36 85.55,49.51 85.55,51.61 J5.36 | U1.K2 69.32,26.57 70.41,26.57 81.86,38.02 81.86,40.72 83.72,42.57 83.72,42.93 84.28,43.48 86,43.48 v86.23,43.26 86.23,42.84 86.55,42.53 U10.64
  Bottom 0.152: R75.1 v84.4,48.36 83.9,48.87 82.02,48.87 81.38,48.23 78.87,48.23 77.78,47.14 77.78,44.09 80.64,41.22 82.37,41.22 83.72,42.57 83.72,42.93 84.28,43.48 86,43.48 v86.23,43.26 C23.1
LCD_DATA11  (via drill 0.3)
  Top 0.152: R57.2 v82.27,48.34 83.01,49.07 83.01,51.61 J5.34 | U1.K1 70.46,27.05 81.56,38.15 81.56,40.92 83.41,42.77 83.41,43.1 84.1,43.79 86.72,43.79 v87.25,43.26 87.78,42.72 88.42,42.72 88.55,42.59 U10.60
  Bottom 0.152: v82.27,48.34 R74.1 80.9,47.42 80.39,47.93 78.99,47.93 78.08,47.02 78.08,44.22 80.77,41.53 82.17,41.53 83.41,42.77 83.41,43.1 84.1,43.79 86.72,43.79 v87.25,43.26 87.76,42.75 C33.1
LCD_DATA12  (via drill 0.3)
  Top 0.152: R56.2 v83.34,48.34 83.34,49.05 J5.35 | U1.L3 68.35,27.53 70.51,27.53 81.25,38.28 81.25,41.05 83.11,42.9 83.11,43.23 83.97,44.09 87.43,44.09 v88.27,43.26 88.37,43.26 89.05,42.58 U10.59
  Bottom 0.152: v83.34,48.34 R73.1 82.93,47.42 82.8,47.3 82.8,46.99 82.7,46.89 81.84,46.89 81.64,47.09 80.8,47.09 80.26,47.62 79.12,47.62 78.38,46.89 78.38,44.35 80.9,41.83 82.04,41.83 83.11,42.9 83.11,43.23 83.97,44.09 87.43,44.09 v88.27,43.26 88.37,43.26 88.77,42.85 C32.1
LCD_DATA13  (via drill 0.3)
  Top 0.152: U1.L2 69.32,27.84 70.38,27.84 80.95,38.41 80.95,41.02 80.42,41.55 v80.42,43.08 R55.2 81.28,43.43 81.43,43.59 83.03,43.59 83.84,44.4 88.06,44.4 v89.2,43.26 89.55,42.91 U10.58 | J5.33 80.29,48.54 80.29,46.71 79.76,46.18 v78.92,46.18
  Bottom 0.152: R72.1 v80.42,43.08 80.11,43.08 78.92,44.27 v78.92,46.18 | C31.1 89.79,42.67 v89.2,43.26
LCD_DATA14  (via drill 0.3)
  Top 0.152: U1.L1 70.43,28.32 80.64,38.53 80.64,40.87 80.06,41.45 80.06,42.55 79.88,42.72 79.88,43.59 v80.37,44.07 R54.2 81.28,44.48 81.38,44.58 81.71,44.58 81.84,44.7 81.84,45.44 81.99,45.59 84.2,45.59 85.09,44.7 88.52,44.7 v89.97,43.26 90.05,43.18 U10.57 | v79.45,47.09 79.45,47.52 79.38,47.6 J5.31
  Bottom 0.152: R71.1 v80.37,44.07 79.73,44.07 79.45,44.35 v79.45,47.09 | C30.1 90.81,42.42 v89.97,43.26
LCD_DATA15  (via drill 0.3)
  Top 0.152: U1.M3 68.35,30.38 70.89,30.38 76.66,36.14 77.32,36.14 79.32,38.15 79.32,44.02 v80.37,45.06 | v80.37,45.06 R53.2 81.28,45.62 81.56,45.9 84.33,45.9 85.22,45.01 90.25,45.01 91.11,44.15 | v92,43.26 91.45,43.8 | 91.45,43.8 91.11,44.15 | U10.56 90.55,42.95 90.5,43 90.5,43.59 90.7,43.79 91.11,43.79 | 91.24,43.79 91.44,43.79 91.45,43.8 | 91.11,44.07 91.11,43.79 | 91.11,43.79 91.24,43.79 | 91.24,43.79 91.24,43.99 91.11,43.99 91.11,44.15 | J5.32 78.31,51.64 78.31,45.77 79.02,45.06 v80.37,45.06
  Bottom 0.152: v80.37,45.06 R70.1 | C29.1 92.38,42.88 v92,43.26
LCD_DE  (via drill 0.3)
  Top 0.152: R28.2 77.27,24.36 77.11,24.51 76.89,24.51 76.71,24.69 76.71,26.36 76.89,26.54 77.75,26.54 78.03,26.82 78.03,28.17 78.97,29.11 81.33,29.11 81.84,29.62 v82.45,29.62 82.83,29.62 83.13,29.31 83.67,29.31 86.06,31.7 87.25,31.7 88.05,32.5 U10.20
  Bottom 0.152: v82.45,29.62 81.84,29.62 81.23,29.01 77.78,29.01 77.62,29.16 77.62,31.19 79.86,33.43 79.86,37.26 79.02,38.1 79.02,41.53 76.86,43.69 76.86,48.03 75.77,49.12 75.77,51.64 J5.30
LCD_HSYNC  (via drill 0.3)
  Top 0.152: R29.2 77.75,25.02 77.98,25.25 77.98,25.86 78.64,26.52 78.64,27.91 79.07,28.35 82.4,28.35 v82.45,28.4 82.83,28.4 83.13,28.7 83.95,28.7 86.33,31.09 87.53,31.09 89.05,32.61 U10.22 | J5.29 76.02,49.35 v76.02,47.6
  Bottom 0.152: v82.45,28.4 77.52,28.4 77.01,28.91 77.01,31.45 79.25,33.68 79.25,37.01 78.41,37.85 78.41,41.27 76.25,43.43 76.25,47.37 v76.02,47.6
LCD_PCLK  (via drill 0.3, 0.3 pad 0.61)
  Top 0.152: U10.4 85.41,40.07 85.34,40.13 84.48,40.13 v84.25,40.36 | v80.85,30.68 80.44,30.28 78.89,30.28 77.27,28.65 R31.2 | J5.28 75.36,51.64 75.36,47.37 75.67,47.07 76.38,47.07 v77.44,48.13
  Bottom 0.152: v84.25,40.36 84.18,40.36 82.68,38.86 81.56,38.86 81.41,38.71 81.41,35.92 81.31,35.81 80.34,35.81 | v80.85,30.68 80.16,31.37 80.16,35.64 | 80.16,35.64 80.16,35.99 | 80.16,35.99 80.16,37.39 79.32,38.23 79.32,41.66 77.17,43.81 77.17,47.85 v77.44,48.13 | 80.16,35.64 80.34,35.81 | 80.34,35.81 80.16,35.99
LCD_VSYNC  (via drill 0.3)
  Top 0.152: R30.2 77.7,26.04 78.33,26.67 78.33,28.04 79.1,28.8 81.56,28.8 81.76,29.01 v81.99,29.01 83.8,29.01 86.18,31.39 87.38,31.39 88.55,32.56 U10.21
  Bottom 0.152: v81.99,29.01 81.76,29.01 81.46,28.7 77.65,28.7 77.32,29.03 77.32,31.32 79.55,33.55 79.55,37.13 78.72,37.97 78.72,41.4 76.56,43.56 76.56,47.9 J5.27
LDO_PGOOD  (via drill 0.3)
  Top 0.152: U1.N4 U1.N5 65.02,30.99 65.51,31.47 65.51,33.91 65.81,34.21 v65.81,35.94
  Bottom 0.152: TP22.TP v65.81,35.94
LED_10_100
  Top 0.152: X5.13 21.77,32.39 22.17,31.98 22.17,24.43 22.35,24.26 28.37,24.26 28.47,24.36 C45.1 R93.1 29.49,25.35 29.5,25.36 U9.24
LED_1000  (via drill 0.3)
  Top 0.152: U9.22 28.7,26.49 28.25,26.04 27.79,26.04 27.46,25.7 R96.2 C44.1 26.44,25.3 v26.16,25.58 | X5.15 21.87,37.47 22.61,36.73 22.61,25.3 22.71,25.2 v22.71,24.79
  Bottom 0.152: v26.16,25.58 25.35,25.58 25.07,25.3 24.08,25.3 23.57,24.79 v22.71,24.79
LED_ACT  (via drill 0.3)
  Top 0.152: U9.21 28.3,26.52 28.12,26.34 27.66,26.34 v26.92,25.6 | C46.1 22.76,22.12 21.89,22.99 X5.11 20.71,22.99 19.43,24.27 19.43,38.12 20.09,38.79 21.46,38.79 22.86,37.39 R104.2
  Bottom 0.152: X5.11 22.15,22.99 23.14,23.98 26.62,23.98 26.92,24.28 v26.92,25.6
MDC
  Top 0.152: U9.40 33.55,31.01 35,31.01 36.55,32.56 36.55,33.58 37.47,34.49 37.47,35.84 37.62,35.99 R139.1
MDIO
  Top 0.152: U9.39 33.52,30.61 33.53,30.61 35.05,30.61 36.85,32.41 36.85,33.45 37.36,33.96 R138.1 R145.2
MDIO_CLK
  Top 0.152: U1.D13 54.08,20.22 54.08,26.04 53.85,26.26 49.38,26.26 48.13,25.02 43.94,25.02 41.78,27.18 41.78,32.56 40.87,33.48 38.71,33.48 38.56,33.63 38.56,35.81 38.73,35.99 R139.2
MDIO_DATA
  Top 0.152: U1.E13 54.38,21.18 54.38,26.16 53.98,26.57 49.25,26.57 48.01,25.32 44.07,25.32 42.09,27.3 42.09,32.69 40.82,33.96 R138.2
MII1_COL  (via drill 0.3)
  Top 0.152: U1.F15 51.84,22.45 50.67,22.45 50.49,22.28 42.95,22.28 42.82,22.4 v42.29,22.4 | R142.2 v25.43,22.94
  Bottom 0.152: v42.29,22.4 41.99,22.4 40.69,21.11 36.35,21.11 35.66,21.79 31.8,21.79 31.22,22.38 25.98,22.38 v25.43,22.94
MII1_RXCLK  (via drill 0.3)
  Top 0.152: R127.2 v39.9,26.85 | v40.41,21.72 40.41,21.39 41.1,20.7 U1.E16
  Bottom 0.152: v39.9,26.85 40.03,26.85 40.41,26.47 v40.41,21.72
MII1_RXD0
  Top 0.152: U1.E14 53.11,20.22 40.18,20.22 38,22.4 37.39,22.4 36.6,23.19 R125.2
MII1_RXD1
  Top 0.152: R122.2 35.59,22.2 36.22,21.57 37.97,21.57 40.11,19.43 U1.D16
MII1_RXD2
  Top 0.152: U1.D15 51.74,19.43 51.18,18.87 40.23,18.87 37.85,21.26 34.11,21.26 33.55,21.82 R121.2
MII1_RXD3  (via drill 0.3)
  Top 0.152: U1.D14 53.11,19.91 40.06,19.91 37.87,22.1 v36.45,22.1 | R120.2 v31.52,22.94
  Bottom 0.152: v31.52,22.94 31.52,22.5 31.93,22.1 v36.45,22.1
MII1_RXDV
  Top 0.152: U1.F16 42.67,21.97 42.57,21.87 41.02,21.87 39.65,23.24 R126.2
MII1_TXCLK
  Top 0.152: U1.H16 50.75,24.51 50.04,23.8 43.43,23.8 42.88,24.36 41.38,24.36 40.87,24.87 40.87,28.35 40.34,28.88 R135.2
MII1_TXD0
  Top 0.152: U1.H15 51.84,24.99 50.8,24.99 49.91,24.11 43.56,24.11 43,24.66 41.5,24.66 41.17,24.99 41.17,29.29 40.56,29.9 R133.2
MII1_TXD1
  Top 0.152: R132.2 40.82,30.91 41.48,30.25 41.48,25.22 41.73,24.97 43.13,24.97 43.69,24.41 49.78,24.41 50.67,25.3 52.22,25.3 53.01,24.51 U1.H14
MII1_TXD2  (via drill 0.3)
  Top 0.152: R131.2 v39.83,31.93 | U1.G16 50.6,23.24 50.24,22.89 43.2,22.89 42.85,23.24 v41.58,23.24
  Bottom 0.152: v39.83,31.93 40.18,31.93 40.72,31.39 40.72,23.65 41.12,23.24 v41.58,23.24
MII1_TXD3  (via drill 0.3)
  Top 0.152: R129.2 v39.85,32.94 | U1.G15 51.84,23.72 50.65,23.72 50.11,23.19 43.33,23.19 42.72,23.8 v42.29,23.8
  Bottom 0.152: v39.85,32.94 40.51,32.94 41.02,32.44 41.02,24.03 41.25,23.8 v42.29,23.8
MII1_TXEN
  Top 0.152: U1.G14 53.01,23.24 52.53,22.76 50.55,22.76 50.37,22.58 43.08,22.58 42.72,22.94 42.04,22.94 41.81,22.71 41.15,22.71 40.56,23.29 40.56,27.33 40.03,27.86 R134.2
MMC0_CD  (via drill 0.3, 0.3 pad 0.61)
  Top 0.152: U1.C14 53.98,18.54 v54.23,18.54 | v89.46,18.87 89.46,20.37 89.94,20.85 v89.94,22.3 | J4.19 v102.23,32.38
  Bottom 0.152: v54.23,18.54 54.23,19.25 54.63,19.66 70.18,19.66 73.84,23.32 77.09,23.32 77.37,23.04 80.19,23.04 81.43,21.79 89.43,21.79 v89.94,22.3 90.35,22.71 90.35,23.22 90.81,23.67 90.81,25.73 91.54,26.47 93.42,26.47 93.83,26.06 95.91,26.06 v102.23,32.38 | X3.CD 91.63,14.38 R92.1 v89.46,18.87
MMC0_CLK  (via drill 0.3, 0.3 pad 0.61)
  Top 0.152: U1.B15 52.32,17.09 v52.76,17.53 | v99.31,17.53 100.71,17.53 101.35,16.89 101.35,15.62 102.62,14.35 R88.1
  Bottom 0.152: v52.76,17.53 52.86,17.63 53.52,17.63 53.75,17.4 55.27,17.4 56.31,18.44 70.69,18.44 74.35,22.1 76.58,22.1 76.86,21.82 79.68,21.82 80.92,20.57 89.79,20.57 90.68,19.68 90.68,19.05 90.99,18.74 X3.5 95.56,18.74 96.77,17.53 v99.31,17.53
MMC0_CMD  (via drill 0.3, 0.3 pad 0.61)
  Top 0.152: U1.B16 v51.69,17.53 | v100.33,18.16 101.09,18.16 101.73,17.53 101.73,16.38 102.74,15.37 R87.1
  Bottom 0.152: v51.69,17.53 52.22,18.06 53.52,18.06 53.87,17.7 55.14,17.7 56.19,18.75 70.56,18.75 74.22,22.4 76.71,22.4 76.99,22.12 79.81,22.12 81.05,20.88 91.69,20.88 X3.3 93.87,20.94 96.65,18.16 v100.33,18.16
MMC0_DAT0  (via drill 0.3, 0.3 pad 0.61)
  Top 0.152: U1.A16 v51.69,16.26 | v100.33,16.89 100.97,16.26 100.97,14.99 102.62,13.34 R89.1
  Bottom 0.152: v51.69,16.26 52.22,16.79 53.06,16.79 53.37,17.09 55.4,17.09 56.44,18.14 70.81,18.14 74.47,21.79 76.45,21.79 76.73,21.51 79.55,21.51 80.8,20.27 89.66,20.27 90.37,19.56 90.37,16.97 90.81,16.54 X3.7 92.59,16.54 92.94,16.89 v100.33,16.89
MMC0_DAT1  (via drill 0.3, 0.3 pad 0.61)
  Top 0.152: U1.A15 52.32,15.82 v52.76,16.26 | R90.1 101.47,12.32 100.58,13.21 100.58,14.99 v99.31,16.26
  Bottom 0.152: v52.76,16.26 52.96,16.26 53.49,16.79 55.52,16.79 56.57,17.83 70.94,17.83 74.6,21.49 76.33,21.49 76.61,21.21 79.43,21.21 80.67,19.96 89.53,19.96 90.07,19.43 90.07,15.98 90.6,15.44 X3.8 94.18,15.44 95,16.26 v99.31,16.26
MMC0_DAT2  (via drill 0.3, 0.3 pad 0.61)
  Top 0.152: U1.C16 51.69,18.8 v52.7,18.8 | v100.33,19.43 101.98,19.43 102.49,18.92 102.49,17.65 102.74,17.4 R86.1
  Bottom 0.152: v52.7,18.8 53.21,18.8 54,18.01 54.46,18.01 54.76,18.31 54.76,19.02 55.09,19.36 70.31,19.36 73.97,23.01 76.96,23.01 77.24,22.73 80.06,22.73 81.31,21.49 89.92,21.49 90.65,22.23 90.65,22.91 90.86,23.11 91.72,23.11 X3.1 92.69,23.14 96.39,19.43 v100.33,19.43
MMC0_DAT3  (via drill 0.3, 0.3 pad 0.61)
  Top 0.152: v55.45,18.82 54.71,18.82 54.46,19.07 53.98,19.07 53.65,18.75 53.44,18.75 52.86,18.16 U1.C15 | v99.31,18.8 101.47,18.8 102.11,18.16 102.11,16.89 102.62,16.38 R91.1
  Bottom 0.152: v55.45,18.82 55.68,19.05 70.43,19.05 74.09,22.71 76.83,22.71 77.11,22.43 79.93,22.43 81.18,21.18 90.07,21.18 90.91,22.02 91.73,22.02 X3.2 93.28,22.04 96.52,18.8 v99.31,18.8
MMC1_CLK  (via drill 0.3)
  Top 0.127: U7.M6 U7.N7 U7.P8
  Top 0.152: J5.21 66.67,50.88 67.08,51.28 72.34,51.28 72.82,50.8 v72.82,48.51 | U1.P2 69.42,32.13 69.9,31.65 70.33,31.65 73.71,35.03 v74.22,35.03 74.75,35.56 74.75,36.07 75.44,36.75 77.01,36.75 78.72,38.46 78.72,41.4 77.52,42.6 U7.P8
  Bottom 0.152: v74.22,35.03 74.75,35.56 74.75,36.93 73.89,37.8 73.89,39.09 70.59,42.39 70.59,44.93 70.94,45.29 71.32,45.29 71.78,45.74 71.78,47.27 71.5,47.55 R51.1 70.97,47.97 71.28,48.28 72.59,48.28 v72.82,48.51
MMC1_CMD  (via drill 0.3, 0.3 pad 0.61)
  Top 0.127: U7.M5 U7.N6 U7.P7
  Top 0.152: U1.P1 70.28,32.31 70.56,32.31 v74.22,35.97 75.31,37.06 76.89,37.06 78.41,38.58 78.41,41.27 77.6,42.09 U7.P7 | J5.20 65.25,51.59 72.69,51.59 73.15,51.13 73.15,49.4 v73.43,49.12
  Bottom 0.152: v74.22,35.97 74.42,36.17 74.42,36.83 73.58,37.67 73.58,38.96 70.28,42.27 70.28,45.06 70.81,45.59 71.2,45.59 71.48,45.87 71.48,46.83 71.3,47 70.13,47 69.98,47.16 R50.1 69.98,47.97 70.65,48.64 72.02,48.64 72.5,49.12 v73.43,49.12
MMC1_DAT0  (via drill 0.3)
  Top 0.152: U1.R3 68.35,34.19 68.35,35.69 69.16,36.5 69.16,38.15 68.86,38.46 v68.86,39.6 69.35,40.09 U7.A3 | J5.25 70.97,50.16 70.66,49.86 70.66,48.78 70.38,48.5 v68,48.5
  Bottom 0.152: v68.86,39.6 68.61,39.85 67.94,39.85 67.16,40.64 67.16,47.19 67.51,47.55 R42.1 v68,48.5
MMC1_DAT1  (via drill 0.3)
  Top 0.152: U1.R2 68.05,32.61 67.39,32.61 67.08,32.92 67.08,33.76 67.36,34.04 67.69,34.04 68.05,34.39 68.05,35.87 68.86,36.68 68.86,38.02 68.25,38.63 v68.25,40.39 68.46,40.59 U7.A4
  Bottom 0.152: v68.25,40.39 67.46,41.17 67.46,46.85 67.61,47 68.83,47 68.99,47.16 R43.1 68.99,48.9 69.19,49.1 70.03,49.1 70.33,49.4 70.33,52.48 70.1,52.7 J5.24
MMC1_DAT2  (via drill 0.3)
  Top 0.152: U1.R1 v69.47,34.04 | v67.72,38.02 67.72,40.74 68.07,41.1 U7.A5 | J5.5 46.35,49.17 47.19,48.34 52.96,48.34 53.9,47.4 54.23,47.4 54.41,47.22 R44.1 54.41,46.35 54.51,46.25 54.74,46.25 54.89,46.1 54.89,45.39 55.32,44.96 58.22,44.96 v58.83,45.57
  Bottom 0.152: v69.47,34.04 69.47,35.66 70.56,36.75 70.56,37.34 70.18,37.72 68.02,37.72 v67.72,38.02 67.46,38.28 65.33,38.28 64.16,39.45 64.16,43 61.59,45.57 v58.83,45.57
MMC1_DAT3  (via drill 0.3, 0.3 pad 0.61)
  Top 0.127: U7.B2 70.51,39.12
  Top 0.152: U1.T3 67.56,36.85 67.79,37.08 v68.33,37.08 | v70,37.08 70.1,37.19 70.1,38.71 U7.A1 70.51,39.12 | v45.29,48.26 45.52,48.03 52.83,48.03 53.37,47.5 R45.1 52.98,46.81 52.76,46.58 52.76,44.65 53.11,44.3 53.9,44.3 54.25,44.65 59.13,44.65 v59.44,44.96
  Bottom 0.152: v70,37.08 v68.33,37.08 68.02,37.39 65.68,37.39 63.86,39.22 63.86,42.72 61.62,44.96 v59.44,44.96 | J5.6 45.29,51.64 v45.29,48.26
MMC1_DAT4  (via drill 0.3)
  Top 0.127: 70.47,39.57 U7.A2 | 70.54,39.65 U7.B3
  Top 0.152: U1.T2 68.83,35.74 69.47,36.37 v69.47,38.81 70.23,39.57 70.47,39.57 | U7.A2 70.54,39.65
  Bottom 0.152: v69.47,38.81 69.22,39.06 68.3,39.06 66.85,40.51 66.85,47.19 66.5,47.55 R46.1 66.02,48.56 66.55,49.1 68.15,49.1 J5.23
MMC1_DAT5  (via drill 0.3)
  Top 0.127: U7.B4 U7.C3 U7.D2 U7.E1 | U7.E1 | U7.E1 72.47,39.11 72.47,39.14 72.49,39.12 U7.E1
  Top 0.152: U1.T1 70.1,36.42 70.92,37.24 v70.92,37.85 71.88,37.85 72.49,38.46 U7.E1
  Bottom 0.152: J5.22 65.89,52.7 65.25,52.07 65.25,48.42 65.02,48.2 R47.1 65.02,47.21 65.23,47 66.4,47 66.55,46.85 66.55,40.39 68.66,38.28 70.48,38.28 v70.92,37.85
MMC1_DAT6  (via drill 0.3)
  Top 0.127: U7.B5 U7.C5 71.6,41.09 71.88,41.38 71.88,42.19 U7.C8 | U7.C8 U7.A10 | U7.C8 | U7.B9 U7.A10 | 70.46,43.61 U7.A10
  Top 0.152: J5.3 43.81,50.98 44.07,51.23 47.02,51.23 47.45,50.8 47.45,49.53 48.34,48.64 53.09,48.64 53.95,47.78 55.14,47.78 55.68,47.24 R48.1 55.68,46.41 55.83,46.25 58.14,46.25 v58.22,46.18 | U1.P4 66.29,32.18 65.81,32.66 65.81,33.73 66.06,33.98 66.4,33.98 66.78,34.37 66.78,36.22 66.32,36.68 v66.32,38.81 66.32,41.07 68.86,43.61 70.46,43.61
  Bottom 0.152: v66.32,38.81 65.46,38.81 64.47,39.8 64.47,43.28 61.57,46.18 v58.22,46.18
MMC1_DAT7  (via drill 0.3)
  Top 0.127: U7.B6 U7.B7 | 70.62,42.46 U7.B7 | 70.62,42.46 U7.A8 | U7.A8 70.62,42.46 | U7.B7
  Top 0.152: U1.R4 67.08,34.19 v67.08,38.81 67.08,41.35 68.28,42.55 69.67,42.55 69.72,42.6 U7.A8 | J5.4 43.81,51.92 44.09,51.64 47.14,51.64 47.75,51.03 47.75,49.76 48.56,48.95 53.21,48.95 54.08,48.08 55.98,48.08 56.69,47.37 R49.1 56.72,46.79 v57.45,46.79
  Bottom 0.152: v57.45,46.79 61.54,46.79 64.77,43.56 64.77,40.46 65.38,39.85 66.6,39.85 67.08,39.37 v67.08,38.81
MON_OUT  (via drill 0.3 pad 0.61)
  Top 0.152: U4.1 46.52,38.22 v46.48,38.25 46.25,38.48 C97.1
  Bottom 0.152: R167.1 45.92,37.69 v46.48,38.25
N$1  (via drill 0.3)
  other vias: 9.78,44.58 9.78,43.81 9.78,43.05
  pour Bottom (no thermals): 3.56,45.54 3.56,44.96 5.46,44.96 6.48,43.94 8,43.94 9.27,42.67 10.29,42.67 10.29,44.96 9.02,44.96 8.64,44.58 6.73,44.58 5.77,45.54
  pour Top (no thermals): 11.43,44.96 11.43,42.67 9.27,42.67 9.27,44.96
N$2
  Top 0.254: D7.2 R38.1
N$3
  Top 0.152: R69.2 98.44,45.71 97.52,44.79 S3.3 98.11,44.13 98.25,44.27 98.25,45.06 98.53,45.34 100.36,45.34 100.81,44.88 100.81,44.22 100.9,44.13 S3.1
N$5  (via drill 0.3 pad 0.61)
  Top 0.152: v23.75,15.88 24.13,15.88 24.65,15.35 U8.34
  Bottom 0.152: v23.75,15.88 24.71,15.88 C101.1 C100.1
N$6  (via drill 0.3)
  Top 0.152: U1.F4 66.75,22.43 v66.75,22.61
  Bottom 0.152: TP1.TP 64.67,23.14 66.45,23.14 66.75,22.84 v66.75,22.61
N$7
  Top 0.152: U8.5 R8.1
N$8
  Top 0.254: D1.2 R26.1
N$9
  Bottom 0.152: U5.1 56.45,29.7 56.26,29.52 56.26,26.62 56.46,26.42 R15.2 56.84,25.91 56.92,25.83 58.57,25.83 58.7,25.7 58.7,25.43 58.8,25.32 R20.1
N$10
  Bottom 0.152: R21.1 60.33,25.73 60.71,26.11 60.71,27.86 60.97,28.13 Q1.B 61.81,28.75 61.54,29.01 60.43,29.01 59.73,29.7 U5.2
N$11
  Top 0.254: D6.2 R37.1
N$13
  Top 0.254: D5.2 R36.1
N$14
  Top 0.152: U8.13 25.15,7.25 TP9.TP
N$15
  Top 0.254: D4.2 R35.1
N$16
  Top 0.152: R102.1 92.76,30.61 93.03,30.34 Y3.3
N$17
  Top 0.152: U8.17 27.18,8.61 27.18,8 27.43,7.75 27.69,7.75 TP10.TP
N$18  (via drill 0.3)
  Top 0.152: U1.G4 66.57,23.24 66.85,23.52 v66.85,23.82
  Bottom 0.152: TP2.TP 64.9,24.38 66.5,24.38 66.85,24.03 v66.85,23.82
N$19  (via drill 0.3)
  Top 0.152: U1.F13 55.14,21.97 v55.5,21.61
  Bottom 0.152: TP3.TP 60.07,21.77 59.69,21.39 55.73,21.39 v55.5,21.61
N$20
  Top 0.152: U1.B4 66.78,16.41 66.78,15.29 67.28,14.78 67.64,14.78 68.45,13.97 R3.1
N$21  (via drill 0.3)
  Top 0.152: U1.G13 54.86,23.55 v55.17,23.85
  Bottom 0.152: TP4.TP 59.05,22.07 58.85,21.87 56.41,21.87 56.19,22.1 56.19,23.47 55.8,23.85 v55.17,23.85
N$22
  Top 0.152: U1.A4 66.29,15.34 67.44,14.2 R4.1
N$23
  Top 0.152: U21.3 38.96,11.81 37.47,10.31 R161.2
N$24  (via drill 0.3)
  Top 0.152: U8.27 29.18,13.43 v29.34,13.59
  Bottom 0.152: R11.1 29.84,13.72 29.72,13.59 v29.34,13.59 28.96,13.59 28.83,13.72 R166.2
N$25
  Top 0.152: U21.7 44.58,13.08 44.45,13.21 44.45,14.73 44.58,14.86 45.11,14.86 45.52,15.27 R160.2
N$26  (via drill 0.3)
  Top 0.152: U1.R13 54.38,33.88 54.38,35.28 55.14,36.04 v55.14,37.21
  Bottom 0.152: R19.1 76.5,36.42 76.17,36.09 76.17,33.63 71.27,28.73 69.39,28.73 69.01,28.35 67.56,28.35 66.65,29.26 65.38,29.26 64.92,29.72 64.92,31.9 62.2,34.62 58.73,34.62 58.12,35.23 58.12,36.4 56.72,37.8 55.35,37.8 55.14,37.59 v55.14,37.21
N$28
  Top 0.152: J10.4 91.21,11.84 94.64,11.84 94.87,12.06 R153.1
N$29
  Top 0.152: R152.1 95.89,11.68 95.73,11.53 93.45,11.53 J10.6
N$30
  Top 0.152: C96.1 46.48,37.47 46.74,37.21 47.3,37.21 U4.3
N$31
  Top 0.152: R151.1 96.9,11.43 95.63,10.16 J10.8
N$32
  Top 0.152: J10.10 97.92,10.92 R150.1
N$33  (via drill 0.3)
  Top 0.152: U1.M16 50.57,29.11 50.11,29.11 49.58,28.57 48.62,28.57 47.88,27.84 45.03,27.84 44.58,27.38 43.76,27.38 43.31,27.84 43.31,31.98 43.54,32.21 v43.54,32.51
  Bottom 0.152: v43.54,32.51 R1.1
N$34
  Top 0.152: Q2.B 72.47,21.75 72.62,21.89 73.05,21.89 73.17,21.77 Q2.C 73.53,21.29 73.69,21.44 73.69,22.12 73.91,22.35 R149.1
N$35
  Top 0.152: J11.1 39.32,7.62 R157.2
N$36
  Top 0.152: U9.1 33.97,31.61 34.37,32 R146.2 34.8,33.71 35,33.91 35,34.98 TP25.P$1
N$38
  Top 0.152: C91.1 87.17,24.16 87.33,24 88.37,24 88.88,24.51 88.88,25.3 88.72,25.45 U23.10
N$42
  Top 0.152: R114.1 73.03,16.84 73.16,16.98 Y5.3
N$47
  Top 0.152: R100.1 23.98,15.24 24.16,15.06 U8.35
N$48  (via drill 0.3)
  Top 0.152: U8.14 v25.65,6.73
  Bottom 0.152: C42.1 C99.1 v25.65,6.73
N$49
  Top 0.152: U10.49 94.05,42.66 94.21,42.82 96.22,42.82 96.8,43.41 96.8,44.78 96.98,44.96 97.13,44.96 97.46,45.29 R118.2
N$53  (via drill 0.3)
  Top 0.152: U1.T12 56.57,35.1 v56.74,35.1
  Bottom 0.152: R23.1 58.06,33.38 57.71,33.73 57.71,34.34 56.95,35.1 v56.74,35.1
N$57
  Top 0.152: U8.11 24.15,8.03 20.56,4.43 D10.1
N$58  (via drill 0.3 pad 0.61)
  Top 0.152: U1.R7 62.76,33.12 v62.76,32.79
  Bottom 0.152: v62.76,32.79 62.76,32 62.46,31.7 61.06,31.7 60.86,31.9 R14.1
N$59
  Top 0.152: D10.2 19.88,2.87 R128.2
N$64
  Top 0.152: X5.12 20.74,24.6 21.64,23.7 R123.2
N$65
  Top 0.152: R124.2 24.89,35.36 24.69,35.56 23.16,35.56 22.91,35.81 22.91,36.85 21.29,38.48 20.3,38.48 19.74,37.92 19.74,35.93 X5.14
N$70
  Top 0.152: U1.F1 70.56,21.97 75.64,27.05 R31.1
N$72  (via drill 0.3)
  Top 0.152: U1.F3 67.89,22.3 v68.2,22.3 | R30.1 75.39,26.04 v74.91,25.55
  Bottom 0.152: v68.2,22.3 71.2,22.3 74.45,25.55 v74.91,25.55
N$77
  Top 0.152: U9.4 30.7,32.58 30.96,32.84 R119.1
N$83
  Top 0.152: U1.F2 69.32,21.49 70.51,21.49 74.04,25.02 R29.1
N$85
  Top 0.152: U1.E1 70.61,20.7 73.86,23.95 76.1,23.95 R28.1
NON_REM0
  Top 0.152: R105.2 29.84,14.1 29.71,14.23 U8.28 27.65,14.7 27.81,14.86 28.07,14.86 28.27,14.66 33.6,14.66 34.52,13.74 34.52,7.11 32.49,5.08 32.49,3.28 TP19.P$1
NON_REM1
  Top 0.152: U8.22 28.9,10.93 28.96,10.87 30.15,10.87 30.61,10.41 30.61,9.65 30.73,9.53 R103.2 31.19,9.14 31.29,9.04 32.84,9.04 33.3,8.59 33.3,7.62 32.79,7.11 31.22,7.11 29.67,5.56 25.55,5.56 24.43,4.45 J8.1
OSC0_GND
  Top 0.203: C7.2 48.26,31.24 48.51,31.5 | 48.51,31.5 48.26,31.75 C12.2 | U1.N15 51.69,31.5 48.51,31.5
OSC0_IN
  Top 0.203: U1.P16 50.04,32.13 49.96,32.05 R32.2 49.28,32.89 48.97,33.2 C12.1 46.3,33.2 Y2.P$2
OSC0_OUT
  Top 0.203: U1.N16 50.04,30.86 49.96,30.94 R32.1 49.28,30.1 48.97,29.79 C7.1 46.3,29.79 Y2.P$1
OSC1_GND
  Top 0.203: U1.B5 64.39,16.26 64.39,15.01 | C5.2 63.8,14.43 64.39,15.01 | C4.2 64.97,14.43 64.39,15.01
OSC1_IN
  Top 0.152: R24.2
  Top 0.203: U1.A6 62.69,14.55 C5.1 62.69,13.61 62.84,13.46 63.63,13.46 63.83,13.26 R24.2 | Y1.P$2 63.14,12.09 63.37,12.32 63.7,12.32 63.83,12.45 R24.2
OSC1_OUT
  Top 0.152: 65.63,12.12 65.64,12.11
  Top 0.203: U1.A5 66.09,14.55 C4.1 66.09,13.61 65.94,13.46 65.15,13.46 64.95,13.26 R24.1 64.95,12.45 65.08,12.32 65.43,12.32 65.63,12.12 | 65.64,12.11 Y1.P$1
PHY_XTAL1
  Top 0.152: Y6.P$2 32.28,35.23 32.08,35.03 C60.1 | C60.1 R117.1 | R119.2 C60.1
PHY_XTAL2
  Top 0.152: U9.5 30.3,33.58 30.18,33.71 R116.1
PHYX
  Top 0.152: Y6.P$1 28.48,35.17 28.63,35.03 C47.1 | R117.2 C47.1 | C47.1 R116.2
PMIC_INT  (via drill 0.3)
  Top 0.152: U1.D4 U1.E4 66.75,21.16 v66.75,21.34
  Bottom 0.152: TP24.TP 64.77,21.64 65.08,21.34 v66.75,21.34
PMIC_MUX_IN  (via drill 0.3)
  Top 0.152: U1.N13 54.38,30.38 v54.38,30.18
  Bottom 0.152: R22.1 R18.2 54.86,29.77 54.81,29.82 54.74,29.82 v54.38,30.18
PMIC_NRESET  (via drill 0.3)
  Top 0.152: U1.M13 54.91,29.64 54.91,30.15 55.35,30.58 55.35,31.06 55.07,31.34 54.48,31.34 54.08,31.75 54.08,32.49 53.95,32.61 53.29,32.61 53.11,32.79 53.11,33.73 52.81,34.04 52.81,34.98 52.25,35.53 51.38,35.53 51.05,35.2 50.7,35.2 v50.62,35.28 | v50.9,36.98 51.05,37.13 51.05,38.25 51.51,38.71 51.51,43.28 50.98,43.81 J2.1
  Bottom 0.152: v50.62,35.28 50.62,35.69 50.9,35.97 v50.9,36.98
PMIC_NWAKEUP  (via drill 0.3)
  Top 0.152: U1.M4 U1.L4 v66.95,27.66
  Bottom 0.152: TP23.TP 66.04,28.57 v66.95,27.66
PMIC_PGOOD  (via drill 0.3)
  Top 0.152: U1.N12 U1.P11 57.02,32.13 56.92,32.23 v56.92,32.79 | U3.2 56.26,41.53 56.39,41.4 56.39,40.77 57.3,39.85 57.3,37.03 55.91,35.64 v55.91,35.38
